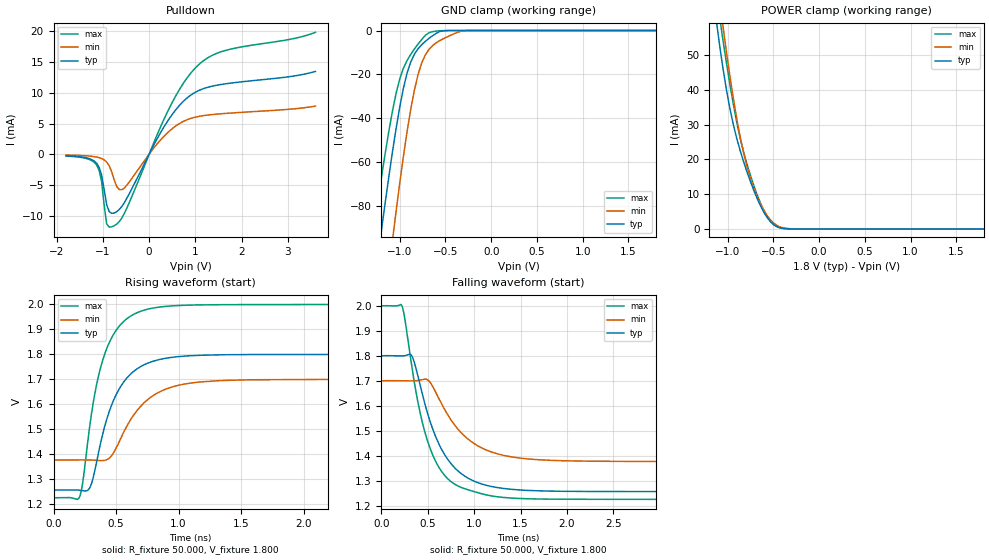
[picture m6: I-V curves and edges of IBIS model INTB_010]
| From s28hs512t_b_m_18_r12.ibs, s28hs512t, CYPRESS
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|   Model INTB_010
[Model] INTB_010
Model_type Open_drain
Polarity   Inverting
Enable   Active-High
Vmeas =  0.900V
Cref =   15.0000pF
Rref =   6.2000k
Vref =   1.8000V
C_comp   5.334pF   5.23pF   5.767pF
[Temperature Range]   25.000   0.125k   -40.000
[Voltage Range]   1.800V   1.700V   2.000V
[Pullup Reference]   1.800V   1.700V   2.000V
[Pulldown Reference]   0.0V   0.0V   0.0V
[POWER Clamp Reference]   1.800V   1.700V   2.000V
[GND Clamp Reference]   0.0V   0.0V   0.0V
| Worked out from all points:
|   slope of the pulldown table from 0 to 0.27 V, typ, clamps not added: 70.9 ohm
|   GND clamp passes 1 mA (typ) near -0.59 V on its own axis
|   POWER clamp passes 1 mA (typ) near -0.48 V on its own axis
|   rising waveform, R_fixture 50.000, V_fixture 1.800: 20-80 % time 221ps typ, 281ps min, 186ps max; typ from 1.26 V to 1.8 V
|   falling waveform, R_fixture 50.000, V_fixture 1.800: 20-80 % time 346ps typ, 420ps min, 288ps max; typ from 1.8 V to 1.26 V
[Pulldown]
|Voltage   I(typ)   I(min)   I(max)
-1.8V     -252.5uA   -134uA     -302.8uA
-1.14V    -1.461mA   -464.4uA   -1.736mA
-1.03V    -3.372mA   -704.8uA   -4.413mA
-920mV    -8.226mA   -1.27mA    -11.35mA
-755mV    -9.59mA    -4.228mA   -11.66mA
-645mV    -8.995mA   -5.77mA    -10.98mA
-535mV    -7.872mA   -5.49mA    -9.628mA
400mV     5.394mA    3.504mA    6.944mA
730mV     8.539mA    5.3mA      11.43mA
1.06V     10.33mA    6.136mA    14.5mA
1.665V    11.48mA    6.65mA     16.93mA
3.6V      13.49mA    7.838mA    19.86mA
[GND_clamp]
|Voltage   I(typ)   I(min)   I(max)
-1.8V     -294mA     -373mA     -247.3mA
-1.28V    -116.8mA   -168.5mA   -89.46mA
-1.2V     -91.34mA   -138.7mA   -67.04mA
-1.08V    -55.6mA    -96.11mA   -36.91mA
-1.04V    -44.83mA   -82.66mA   -28.74mA
-1V       -34.98mA   -69.76mA   -22.14mA
-920mV    -19.48mA   -46.23mA   -13.73mA
-800mV    -8.377mA   -20.18mA   -6.205mA
-680mV    -3.579mA   -8.59mA    -1.029mA
-560mV    -408.3uA   -4.544mA   -113.8uA
-280mV    -162.8nA   -73.51uA   -82.13nA
1.8V      272.8pA    325nA      188.3pA
[POWER_clamp]
|Voltage   I(typ)   I(min)   I(max)
-1.8V     236.7mA    239.1mA    251.1mA
-1.123V   59.68mA    73.25mA    67.66mA
-1.086V   52.46mA    65.42mA    60.6mA
-1.049V   45.83mA    57.89mA    53.9mA
-938mV    30.03mA    37.57mA    35.87mA
-864mV    22.62mA    26.6mA     26.18mA
-790mV    16.52mA    18.14mA    18.76mA
-716mV    11.21mA    11.92mA    12.63mA
-642mV    6.708mA    7.258mA    7.47mA
-494mV    1.178mA    1.619mA    1.205mA
-272mV    6.291uA    28.11uA    4.439uA
1.8V      0A         0A         0A
[Ramp]
| variable   typ   min   max
dV/dt_r   0.332/0.363n   0.244/0.435n   0.460/0.300n
dV/dt_f   0.326/0.346n   0.194/0.419n   0.465/0.288n
R_load = 50.000
[Rising Waveform]
R_fixture= 50.000
V_fixture= 1.800
V_fixture_min= 1.700
V_fixture_max= 2.000
|time   V(typ)   V(min)   V(max)
0s        1.256V     1.377V     1.225V
205ps     1.256V     1.377V     1.226V
232ps     1.254V     1.377V     1.282V
297ps     1.273V     1.377V     1.537V
345ps     1.37V      1.375V     1.68V
414ps     1.519V     1.376V     1.808V
564ps     1.691V     1.491V     1.933V
754ps     1.765V     1.619V     1.981V
1.337ns   1.798V     1.695V     1.999V
6ns       1.8V       1.7V       2V
[Falling Waveform]
R_fixture= 50.000
V_fixture= 1.800
V_fixture_min= 1.700
V_fixture_max= 2.000
|time   V(typ)   V(min)   V(max)
0s        1.8V       1.7V       2V
217ps     1.799V     1.7V       2.002V
335ps     1.794V     1.699V     1.74V
415ps     1.686V     1.702V     1.575V
509ps     1.555V     1.7V       1.446V
679ps     1.406V     1.586V     1.322V
899ps     1.318V     1.477V     1.268V
1.179ns   1.277V     1.416V     1.239V
1.684ns   1.259V     1.384V     1.227V
6ns       1.256V     1.377V     1.225V
